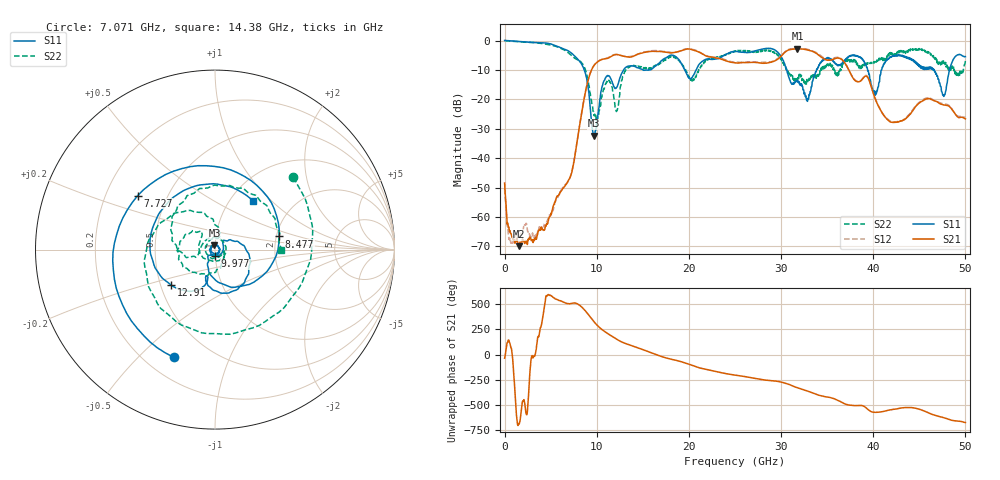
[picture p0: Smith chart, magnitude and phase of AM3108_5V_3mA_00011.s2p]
# Hz S DB R 50.0
!freq dBS11 angS11 dBS21 angS21 dBS12 angS12 dBS22 angS22
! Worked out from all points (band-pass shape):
!   1601 points, 10 MHz to 50 GHz, reference 50 ohm
!   highest |S21| = -2.80 dB at 31.78 GHz (marker M1); lowest = -69.9 dB at 1.603 GHz (marker M2)
!   |S21| within 3 dB of the highest: 11.35 GHz to 22.81 GHz (11.45 GHz wide, 67.1 % of centre); 29.85 GHz to 34.44 GHz (4.585 GHz wide, 14.3 % of centre)
!   lowest |S11| = -32.4 dB at 9.664 GHz (marker M3), VSWR 1.05, Z = 49.6 + j2.36 ohm
!   |S11| at or under -10 dB: 8.657 GHz to 12.92 GHz (4.266 GHz wide, 39.5 % of centre); 30.62 GHz to 33.84 GHz (3.224 GHz wide, 10 % of centre); 46.63 GHz to 48.29 GHz (1.662 GHz wide, 3.5 % of centre)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
!   |S22| runs from -27.4 to 0.0 dB; largest |S21 - S12| = 0.027
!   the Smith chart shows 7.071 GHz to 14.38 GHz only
!   S11 on the Smith chart (normalised r, x): 7.071 GHz: 0.31, -0.64; 7.727 GHz: 0.34, +0.28; 8.477 GHz: 2.07, +0.35; 9.977 GHz: 1.00, -0.07; 12.91 GHz: 0.57, -0.25; 14.38 GHz: 1.27, +0.79
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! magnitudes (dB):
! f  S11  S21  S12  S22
! 10 MHz  0.0  -48.5  -50.3  0.0
! 666.1 MHz  -0.1  -65.5  -68.7  -0.2
! 1.603 GHz  -0.3  -69.9  -66.2  -0.5
! 7.071 GHz  -3.8  -46.8  -47.0  -4.5
! 7.727 GHz  -5.6  -37.4  -37.3  -6.2
! 8.352 GHz  -8.0  -25.0  -24.8  -7.5
! 8.477 GHz  -8.8  -22.6  -22.5  -7.9
! 9.664 GHz  -32.4  -8.7  -8.7  -24.1
! 9.977 GHz  -28.5  -7.5  -7.5  -27.4
! 10.91 GHz  -12.9  -6.2  -6.2  -15.5
! 12.16 GHz  -16.0  -4.8  -4.7  -24.0
! 12.91 GHz  -10.0  -5.3  -5.3  -11.5
! 14.38 GHz  -9.2  -4.7  -4.7  -8.7
! 16.69 GHz  -7.9  -3.7  -3.5  -8.3
! 25 GHz  -3.7  -7.6  -7.3  -3.7
! 31.78 GHz  -14.1  -2.8  -2.7  -13.6
! 33.35 GHz  -15.4  -3.6  -3.5  -12.7
! 38 GHz  -5.0  -13.5  -13.4  -6.6
! 40.22 GHz  -18.6  -19.9  -19.6  -7.6
! 41.69 GHz  -6.0  -27.3  -27.0  -5.2
! 47.66 GHz  -19.0  -21.9  -21.5  -7.8
! 50 GHz  -5.5  -26.6  -26.2  -6.8
